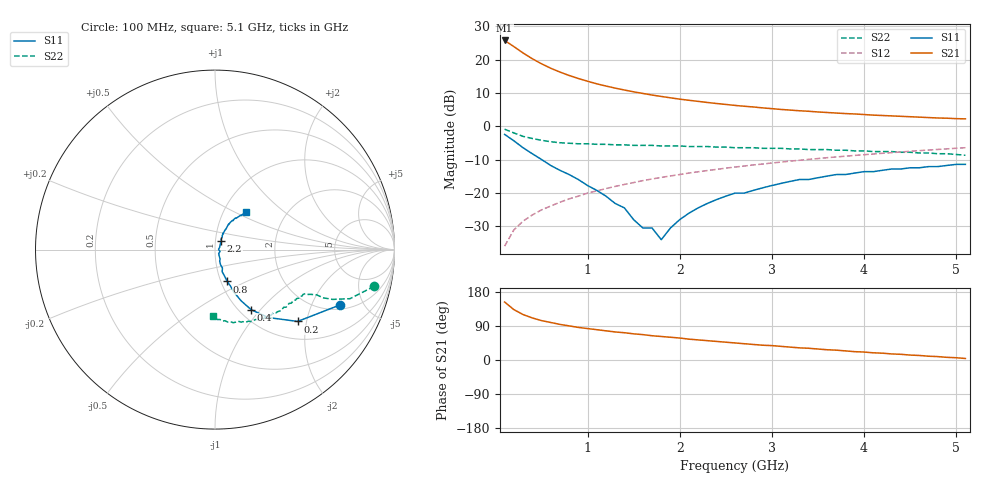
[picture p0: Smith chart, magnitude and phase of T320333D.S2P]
!AT-32033
!S PARAMETERS at Vce=2.7V  Ic=7.5mA.  LAST UPDATED 01-05-95
# ghz s ma r 50
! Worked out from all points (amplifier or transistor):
!   51 points, 100 MHz to 5.1 GHz, reference 50 ohm
!   highest |S21| = 25.8 dB at 100 MHz (marker M1)
!   |S21| within 3 dB of that: start of sweep to 260.9 MHz
!   unconditionally stable (mu >= 1): 1.088 GHz to 2.292 GHz; 2.308 GHz to 2.452 GHz; 2.595841 GHz to 2.603623 GHz
!   at 900 MHz: K = 0.98, MSG = 17.7 dB, |S12| = -20.9 dB
!   at 2.6 GHz: K = 1.00, MAG = 9.2 dB, |S12| = -12.2 dB
!   at 5.1 GHz: K = 0.93, MSG = 4.3 dB, |S12| = -6.4 dB
!   S11 on the Smith chart (normalised r, x): 100 MHz: 2.23, -3.27; 200 MHz: 1.39, -1.77; 400 MHz: 1.13, -0.89; 800 MHz: 1.07, -0.39; 2.2 GHz: 1.06, +0.11; 5.1 GHz: 1.28, +0.57
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0.1  0.76 -24.0  19.51 153.0  0.016 78.0  0.91 -13.0
0.2  0.61 -41.0  15.8 133.0  0.028 72.0  0.8 -20.0
0.3  0.48 -52.0  12.67 120.0  0.038 70.0  0.71 -23.0
0.4  0.39 -59.0  10.38 111.0  0.047 70.0  0.66 -24.0
0.5  0.32 -63.0  8.72 104.0  0.056 69.0  0.62 -24.0
0.6  0.26 -66.0  7.48 99.0  0.064 69.0  0.59 -25.0
0.7  0.22 -67.0  6.55 94.0  0.073 70.0  0.57 -26.0
0.8  0.19 -69.0  5.82 90.0  0.082 70.0  0.56 -26.0
0.9  0.16 -70.0  5.24 86.0  0.09 69.0  0.55 -27.0
1  0.13 -72.0  4.77 83.0  0.1 69.0  0.55 -28.0
1.1  0.11 -68.0  4.36 80.0  0.108 69.0  0.54 -29.0
1.3  0.07 -68.0  3.76 74.0  0.126 68.0  0.53 -31.0
1.5  0.04 -55.0  3.31 69.0  0.144 66.0  0.52 -33.0
1.6  0.03 -47.0  3.13 67.0  0.154 66.0  0.52 -34.0
1.7  0.03 -21.0  2.96 64.0  0.163 65.0  0.52 -35.0
1.8  0.02 5.0  2.82 62.0  0.172 64.0  0.51 -36.0
2  0.04 44.0  2.57 58.0  0.19 62.0  0.51 -39.0
2.2  0.06 56.0  2.38 53.0  0.209 61.0  0.5 -42.0
2.6  0.1 62.0  2.07 45.0  0.246 57.0  0.48 -47.0
3.5  0.17 61.0  1.65 29.0  0.33 48.0  0.45 -62.0
4.3  0.23 54.0  1.44 16.0  0.405 39.0  0.42 -76.0
5.1  0.27 50.0  1.3 4.0  0.48 30.0  0.37 -92.0
